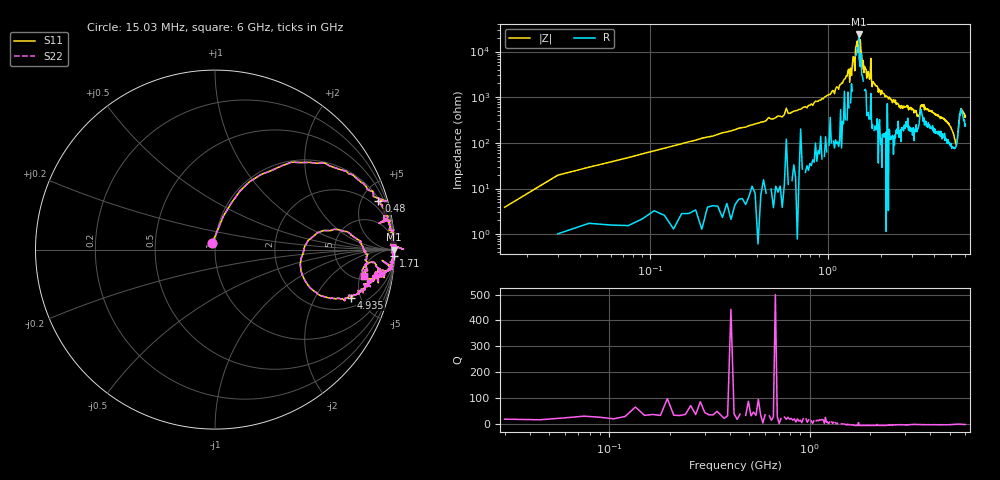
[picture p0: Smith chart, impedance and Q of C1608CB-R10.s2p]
!	Network	Analyzer	HP8753E.07.74:	Oct	30	2002	Serial	No.	JP38451487
!	Hewlett-Packard
!	7	Sep	2009	9:53:08
!	Frequency	S11	S21	S12	S22
#	HZ	S	RI	R	50
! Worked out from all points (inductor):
!   400 points, 15.03 MHz to 6 GHz, reference 50 ohm
!   read as one part in series: L = 102 nH near 45.03 MHz
!   highest |Z| = 23.7 kohm at 1.5 GHz (marker M1)
!   self-resonance near 1.485 GHz
!   S11 on the Smith chart (normalised r, x): 15.03 MHz: 0.97, +0.07; 480 MHz: 1.19, +6.63; 1.71 GHz: 8, -59; 4.935 GHz: 2.72, -4.14; 6 GHz: 5.70, -5.87
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1.502992e7  -0.0146 0.0374  1.01 -0.0374  1.01 -0.0374  -0.0146 0.0374
3.002985e7  0.0459 0.185  0.954 -0.185  0.954 -0.185  0.0459 0.185
1.050295e8  0.318 0.442  0.682 -0.442  0.682 -0.442  0.318 0.442
4.800276e8  0.91 0.272  0.0901 -0.272  0.0901 -0.272  0.91 0.272
1.020025e9  0.986 0.0843  0.0138 -0.0843  0.0138 -0.0843  0.986 0.0843
1.320023e9  0.996 0.0238  0.00403 -0.0238  0.00403 -0.0238  0.996 0.0238
1.335023e9  1.05 0.00122  -0.0495 -0.00122  -0.0495 -0.00122  1.05 0.00122
1.425023e9  1 0.0264  -0.00048 -0.0264  -0.00048 -0.0264  1 0.0264
1.500022e9  0.996 -0.000946  0.00409 0.000946  0.00409 0.000946  0.996 -0.000946
1.515022e9  0.985 -0.0036  0.0146 0.0036  0.0146 0.0036  0.985 -0.0036
1.530022e9  0.999 -0.00528  0.00143 0.00528  0.00143 0.00528  0.999 -0.00528
1.575022e9  0.983 -0.0167  0.0166 0.0167  0.0166 0.0167  0.983 -0.0167
1.710021e9  0.995 -0.0329  0.00482 0.0329  0.00482 0.0329  0.995 -0.0329
1.755021e9  0.997 0.0138  0.00259 -0.0138  0.00259 -0.0138  0.997 0.0138
1.785021e9  0.99 -0.0573  0.0104 0.0573  0.0104 0.0573  0.99 -0.0573
2.01002e9  0.989 -0.0701  0.0113 0.0701  0.0113 0.0701  0.989 -0.0701
3.015015e9  0.931 -0.152  0.0689 0.152  0.0689 0.152  0.931 -0.152
4.00501e9  0.885 -0.173  0.115 0.173  0.115 0.173  0.885 -0.173
4.935005e9  0.76 -0.267  0.24 0.267  0.24 0.267  0.76 -0.267
5.010005e9  0.728 -0.27  0.272 0.27  0.272 0.27  0.728 -0.27
5.460003e9  0.664 0.113  0.336 -0.113  0.336 -0.113  0.664 0.113
6e9  0.831 -0.148  0.169 0.148  0.169 0.148  0.831 -0.148
